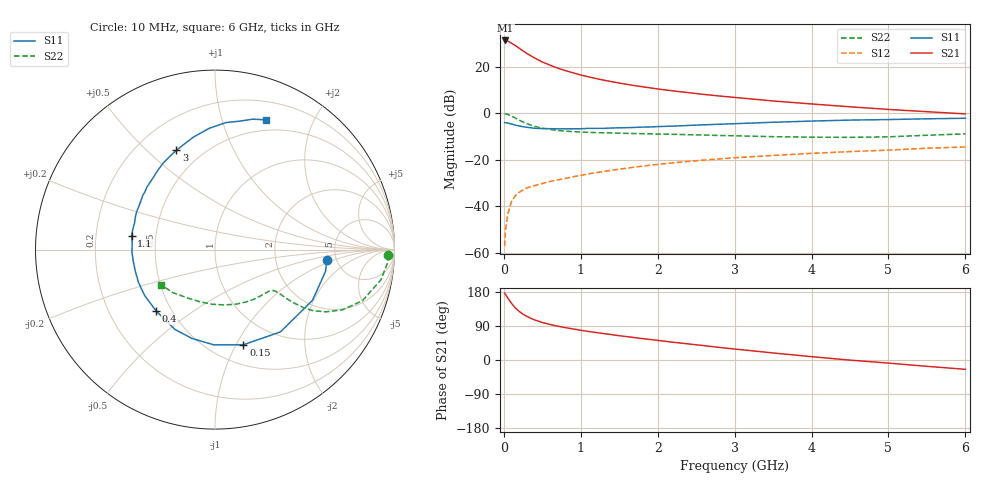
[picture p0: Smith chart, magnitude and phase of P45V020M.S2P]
! SIEMENS Small Signal Semiconductors
! BFP182
! Si NPN RF Bipolar Junction Transistor in SOT143
! VCE = 5 V  IC = 20 mA
! Common Emitter S-Parameters:  March  1996
# GHz  S  MA  R  50
!  f  S11  S21  S12  S22
! GHz  MAG  ANG  MAG  ANG  MAG  ANG  MAG  ANG
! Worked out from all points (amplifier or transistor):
!   36 points, 10 MHz to 6 GHz, reference 50 ohm
!   highest |S21| = 31.2 dB at 20 MHz (marker M1)
!   |S21| within 3 dB of that: start of sweep to 185.2 MHz
!   unconditionally stable (mu >= 1): 842.7 MHz to 5.42 GHz
!   at 250 MHz: K = 0.47, MSG = 29.8 dB, |S12| = -33.0 dB
!   at 1.4 GHz: K = 1.13, MAG = 16.8 dB, |S12| = -24.5 dB
!   at 6 GHz: K = 0.95, MSG = 7.1 dB, |S12| = -14.5 dB
!   S11 on the Smith chart (normalised r, x): 10 MHz: 4.18, -0.78; 150 MHz: 0.70, -1.07; 400 MHz: 0.41, -0.36; 1.1 GHz: 0.36, +0.07; 3 GHz: 0.36, +0.62; 6 GHz: 0.38, +1.40
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0.01  0.6249 -5.2  36.05 176.3  0.0014 82.3  0.9661 -1.8
0.02  0.6279 -11.0  36.28 173.5  0.003 86.6  0.966 -4.1
0.05  0.6123 -27.5  35.2 163.7  0.0068 78.8  0.9399 -10.3
0.1  0.5859 -51.5  31.73 149.5  0.0127 67.4  0.8695 -19.1
0.15  0.5534 -73.4  28.19 137.4  0.017 60.6  0.7853 -25.3
0.2  0.5306 -90.7  24.7 128.1  0.0201 56.8  0.7084 -29.3
0.25  0.5114 -104.5  21.55 120.7  0.0225 54.5  0.6445 -31.9
0.3  0.4978 -116.6  19.08 115.0  0.025 51.8  0.5937 -33.2
0.4  0.474 -133.8  15.25 105.7  0.0279 50.6  0.5211 -34.2
0.5  0.4682 -146.9  12.53 99.1  0.031 50.1  0.4755 -34.4
0.6  0.4639 -156.7  10.72 93.8  0.0342 50.9  0.4468 -34.3
0.7  0.46 -165.4  9.224 89.3  0.0369 51.5  0.4257 -34.3
0.9  0.4628 -178.4  7.32 82.0  0.0432 52.7  0.4012 -34.8
1.1  0.4714 170.6  6.031 75.3  0.0499 53.2  0.3872 -36.3
1.5  0.4847 154.3  4.432 64.1  0.0628 52.5  0.3722 -40.5
1.8  0.5023 143.4  3.69 56.5  0.0728 51.4  0.3627 -44.8
2.2  0.5272 131.3  3.005 46.9  0.0859 48.9  0.352 -51.6
3  0.594 111.2  2.176 29.0  0.1104 42.2  0.3271 -68.1
3.5  0.6377 101.0  1.826 18.6  0.1237 37.7  0.3129 -80.2
4.5  0.71 85.2  1.369 -0.3  0.1498 29.1  0.3026 -107.3
5.5  0.7563 73.9  1.075 -16.7  0.177 21.2  0.3357 -134.4
6  0.7773 68.5  0.964 -24.6  0.1883 16.3  0.3594 -147.1
